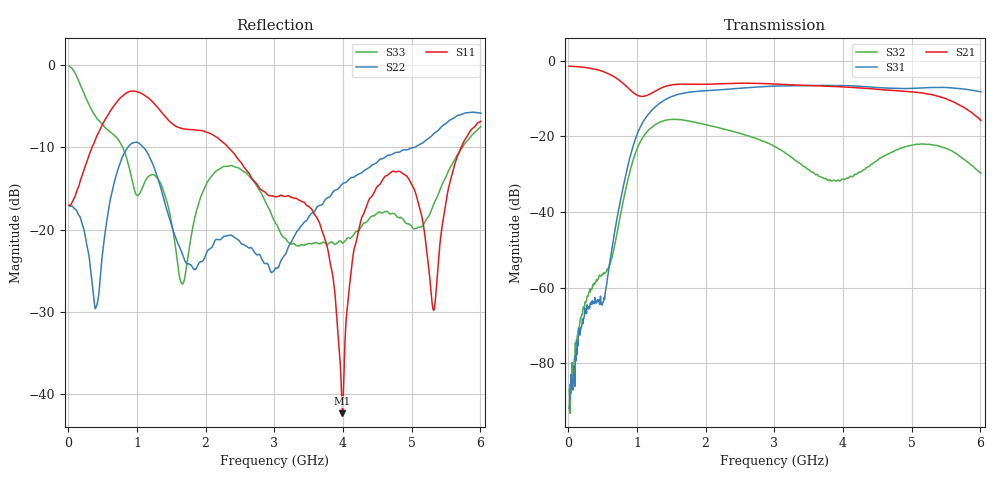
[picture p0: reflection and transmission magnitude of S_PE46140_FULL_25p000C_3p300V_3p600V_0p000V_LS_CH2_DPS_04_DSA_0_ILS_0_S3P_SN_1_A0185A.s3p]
! Device ID: PE46140_FULL
! File Path: z:\PE46140\MajorStates\25p000C\3p300\LS_CH2_DPS_04_DSA_0_ILS_0\PE46140_FULL_25p000C_3p300V_3p600V_0p000V_LS_CH2_DPS_04_DSA_0_ILS_0_S3P_SN_1_A0185A.s3p
! Serial: 1
! Lot: A0185A
! Temp: 25.000C
! VDD: 3.300
! VSS: 0.000
! Control_Hi: 3.600
! Control_Lo: 0.000
! Logic State: LS_CH2_DPS_04_DSA_0_ILS_0
! Port 1: RFIN
! Port 2: RFOUT1
! Port 3: RFOUT2
! ThroughPath:1-3
! IDD: 0.0003146954
! ISS: -2.366e-007
! Comment:
#  Hz  S  RI  R  50
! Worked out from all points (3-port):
!   801 points, 10 MHz to 6.01 GHz, reference 50 ohm
!   strongest paths, dB at 10 MHz, 1.51 GHz, 3.01 GHz, 4.51 GHz, 6.01 GHz:
!     S21: -1.5, -6.4, -6.2, -7.6, -15.8
!     S31: -91.9, -9.5, -6.8, -7.2, -8.3
!     S32: -86.9, -15.6, -22.8, -26.2, -29.8
!   lowest |S11| = -42.3 dB at 3.993 GHz (marker M1), VSWR 1.02, Z = 50.5 - j0.572 ohm
!   |S11| at or under -10 dB: start of sweep to 346.2 MHz; 2.324 GHz to 5.724 GHz (3.401 GHz wide, 84.5 % of centre)
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1e7  0.1401 -0.0109  0.8419 -0.0244  1.93e-05 -1.07e-05
     0.8418 -0.0243  0.1399 -0.00682  -5.67e-05 -3.1e-05
     -1.95e-05 1.63e-05  4.51e-05 -4.11e-06  0.9748 -0.093
3.55e8  -0.016 -0.3218  0.4591 -0.6282  -0.00058 -0.00036
        0.4592 -0.6262  -0.00904 -0.0427  -0.000105 0.00107
        -0.000542 -0.000296  -8.62e-05 0.00109  -0.46 -0.2356
1.165e9  -0.5865 0.2267  -0.2031 -0.2873  -0.1947 -0.0177
         -0.2032 -0.2879  0.2135 -0.1883  0.00384 0.1196
         -0.195 -0.0181  0.00367 0.1196  0.1772 0.112
1.9525e9  -0.1991 0.3445  -0.4305 0.224  0.3914 -0.0639
          -0.4307 0.2239  0.0597 -0.0241  -0.1437 -0.0213
          0.3916 -0.0639  -0.1439 -0.0214  0.0552 0.1578
3.01e9  0.0178 0.1569  0.4075 0.2705  -0.4289 -0.1636
        0.4072 0.2714  -0.0574 -0.00136  0.0587 -0.0426
        -0.4292 -0.1641  0.0587 -0.0426  0.1001 -0.048
3.67e9  0.0422 0.0975  0.3448 -0.3057  -0.241 0.4016
        0.3453 -0.3053  0.0491 0.1314  -0.0248 0.0149
        -0.2413 0.402  -0.0249 0.0151  0.0819 0.000196
3.9925e9  0.00519 -0.00566  0.0823 -0.4405  0.0552 0.4638
          0.0829 -0.4402  0.1323 0.1346  0.0224 0.0156
          0.0554 0.4637  0.0222 0.0156  0.0827 0.00301
4.3825e9  -0.1273 -0.0842  -0.2528 -0.3422  0.348 0.2815
          -0.2527 -0.3428  0.216 0.099  0.00415 -0.0396
          0.3485 0.2809  0.00442 -0.0398  0.1152 -0.0143
5.32e9  -0.0224 -0.0234  -0.1256 0.3259  0.2261 -0.3781
        -0.1267 0.3261  0.3785 -0.0356  0.0294 0.0706
        0.2264 -0.3778  0.0292 0.0708  0.1319 0.0513
6.01e9  -0.3102 -0.3296  0.1546 0.0472  -0.2933 -0.2497
        0.1548 0.0475  0.2471 -0.4429  0.0193 -0.0259
        -0.2949 -0.2501  0.0192 -0.0262  0.4195 0.0292
